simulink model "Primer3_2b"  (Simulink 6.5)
settings: Solver=ode23t  SolverMode=SingleTasking  StartTime=0.0  StopTime=0.6  RelTol=1e-3  AbsTol=1e-6
undefined symbols (not defined in the file or in its folder): blocks, Continuous, powergui, ZData
libraries: powerlib x14

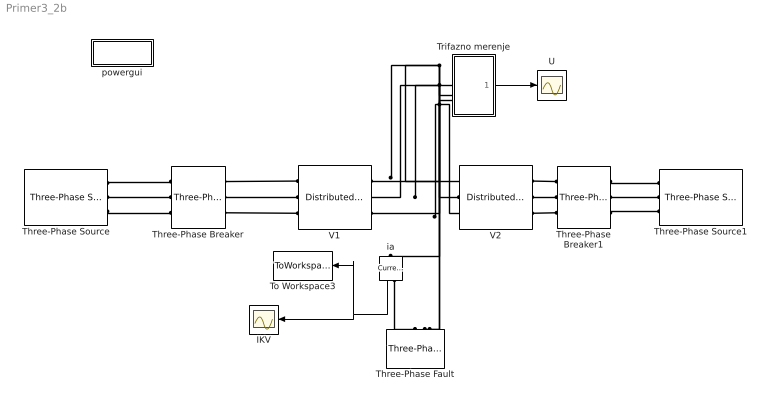
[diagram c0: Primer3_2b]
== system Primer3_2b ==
  IKV : Scope
  Three-Phase Breaker : powerlib/Elements/Three-Phase Breaker  DialogController=PMDialogs.PMDefaultMaskDlg  SystemSampleTime=-1  InitialState=closed  SwitchA=on  SwitchB=off  SwitchC=off  SwitchTimes="[ 10/50  20/50 ]"  External=off  BreakerResistance=0.001  SnubberResistance=1e6  SnubberCapacitance=inf  Measurements=None
  Three-Phase Breaker1 : powerlib/Elements/Three-Phase Breaker  Orientation=left  DialogController=PMDialogs.PMDefaultMaskDlg  SystemSampleTime=-1  InitialState=closed  SwitchA=on  SwitchB=off  SwitchC=off  SwitchTimes="[ 10/50  20/50 ]"  External=off  BreakerResistance=0.001  SnubberResistance=1e6  SnubberCapacitance=inf  Measurements=None
  Three-Phase Fault : powerlib/Elements/Three-Phase Fault  Orientation=down  DialogController=PMDialogs.PMDefaultMaskDlg  SystemSampleTime=-1  FaultA=on  FaultB=off  FaultC=off  FaultResistance=0.001  GroundFault=on  GroundResistance=0.001  External=off  SwitchStatus=[1 0]  SwitchTimes=[ 3/50 15/50]  InitialStates=[0 0 1]  SnubberResistance=1e6  SnubberCapacitance=inf  Measurements=None
  Three-Phase Source : powerlib/Electrical Sources/Three-Phase Source  DialogController=PMDialogs.PMDefaultMaskDlg  SystemSampleTime=-1  Voltage=410e3  PhaseAngle=0  Frequency=50  InternalConnection=Yg  SpecifyImpedance=on  Resistance=0.8929  Inductance=16.58e-3  ShortCircuitLevel=sqrt(3)*400e3*16e3  BaseVoltage=400e3  XRratio=10
  Three-Phase Source1 : powerlib/Electrical Sources/Three-Phase Source  Orientation=left  DialogController=PMDialogs.PMDefaultMaskDlg  SystemSampleTime=-1  Voltage=395e3  PhaseAngle=-2.5  Frequency=50  InternalConnection=Yg  SpecifyImpedance=on  Resistance=0.8929  Inductance=16.58e-3  ShortCircuitLevel=sqrt(3)*400e3*14e3  BaseVoltage=400e3  XRratio=10
  To Workspace3 : ToWorkspace  VariableName=ikv  SampleTime=-1  SaveFormat=Array
  Trifazno merenje : Subsystem
  U : Scope
  V1 : powerlib/Elements/Distributed Parameters Line  DialogController=PMDialogs.PMDefaultMaskDlg  SystemSampleTime=-1  Phases=3  Frequency=50  Resistance=[0.029983 0.29405]  Inductance=[0.0010055 0.0025377]  Capacitance=[1.1784e-008 8.6541e-009]  Length=113.5/2  x1=[0 5.31470182416808e-011 178450.018618737 -366847.020662789;5.31896283741607e-005 5.41899780765739e-011 184554.839172681 -363814.04185674;0.000106379256748321 5.5217807089294e-011 190608.12867694 -360679.479588827;0.000159568885122482 5.62302182913874e-011 196608.19694358 -357444.209085539;0.000212758513496643 5.72269289993319e-011 202553.368645001 -354109.133692926;0.000265948141870804 5.82076609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  x2=[0 -3.7359824086561e-011 172736.109706228 -365994.140775089;5.31896283741607e-005 -4.15549298166249e-011 178827.477001409 -363056.756096685;0.000106379256748321 -4.57384326585573e-011 184868.912430032 -360017.999404301;0.000159568885122482 -4.99091645026855e-011 190858.729114034 -356878.719173774;0.000212758513496643 -5.40659608052301e-011 196795.254588242 -353639.791948936;0.000265948141870804 -5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  x3=[0 6.15163419918279e-012 586.956046574621 -949.442634179271;5.31896283741607e-005 6.07772862185656e-012 602.738564141177 -939.502495741663;0.000106379256748321 6.00212603275329e-012 618.352786197114 -929.300031211689;0.000159568885122482 5.92484754148351e-012 633.794352969173 -918.838089302008;0.000212758513496643 5.84591472559994e-012 649.058952892574 -908.119591176059;0.000265948141870804 5.7653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  x4=[0 -5.27235691341477e-012 533.264836498699 -1585.21009257672;5.31896283741607e-005 -5.22831622679303e-012 559.67803894775 -1576.07833440241;0.000106379256748321 -5.18281569970079e-012 585.934969163778 -1566.50650664595;0.000159568885122482 -5.1358680367083e-012 612.028295736881 -1556.49728193482;0.000212758513496643 -5.08748634645237e-012 637.950732938252 -1546.05345502561;0.000265948141870804 -5.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  x5=0.000265948141870804  Measurements=None
  V2 : powerlib/Elements/Distributed Parameters Line  DialogController=PMDialogs.PMDefaultMaskDlg  SystemSampleTime=-1  Phases=3  Frequency=50  Resistance=[0.029983 0.29405]  Inductance=[0.0010055 0.0025377]  Capacitance=[1.1784e-008 8.6541e-009]  Length=113.5/2  x1=[0 -3.7359824086561e-011 172736.109706228 -365994.140775089;5.31896283741607e-005 -4.15549298166249e-011 178827.477001409 -363056.756096685;0.000106379256748321 -4.57384326585573e-011 184868.912430032 -360017.999404301;0.000159568885122482 -4.99091645026855e-011 190858.729114034 -356878.719173774;0.000212758513496643 -5.40659608052301e-011 196795.254588242 -353639.791948936;0.000265948141870804 -5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  x2=[0 -1.00365319719216e-010 166509.443707765 -363699.090775954;5.31896283741607e-005 -9.78077225317173e-011 172563.331767605 -360866.069344832;0.000106379256748321 -9.52228156587506e-011 178569.037023553 -357932.287579098;0.000159568885122482 -9.26113208530759e-011 184524.882574059 -354898.564643695;0.000212758513496643 -8.99739672912847e-011 190429.205439304 -351765.747608946;0.000265948141870804 -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  x3=[0 -9.13979376899358e-012 644.436346866573 -910.109116757214;5.31896283741607e-005 -9.09687067248558e-012 659.553606600837 -899.214017677193;0.000106379256748321 -9.05140756512387e-012 674.486707036846 -888.067841776699;0.000159568885122482 -9.00341714103046e-012 689.231478582818 -876.673701269678;0.000212758513496643 -8.9529127999999e-012 703.783804231807 -865.034777606277;0.000265948141870804 -8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  x4=[0 8.15651641056055e-012 435.415414146165 -1612.56297375389;5.31896283741607e-005 8.11939388275095e-012 462.299323032324 -1605.06238605293;0.000106379256748321 8.08000427328985e-012 489.05414958452 -1597.11363589828;0.000159568885122482 8.03835858046876e-012 515.672423371187 -1588.71894272478;0.000212758513496643 7.9944684325185e-012 542.146712088759 -1579.88065048263;0.000265948141870804 7.948346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  x5=0.000265948141870804  Measurements=None
  ia : powerlib/Measurements/Current Measurement  Orientation=down  DialogController=PMDialogs.PMDefaultMaskDlg  SystemSampleTime=-1  PhasorSimulation=off  OutputType=Complex  PSBequivalent=0
  powergui : Subsystem  AncestorBlock=powerlib/powergui  InitFcn=powergui( 'InitFcn_Callback' , gcb , 0 , [ ] );  mask(PSB option menu block){SimulationMode=Continuous, SampleTime=50e-6, echomessages=off, RestoreLinks=warning, x0status=blocks, Frange=[0:2:500], Ylog=off, Xlog=on, ShowGrid=off, save=off, variable=ZData, structure=, ZoomFFT=on, StartTime=0.0, cycles=1, DisplayStyle=1, fundamental=60, FreqAxis=off, MaxFrequency=1000, frequencyindice=50, frequencyindicesteady=1, RmsSteady=1, display=off, Ts=0, frequency=60, methode=off, HookPort=off, Interpol=off}
      mask prompts: SimulationMode "Simulation mode"; SampleTime "Sample time Ts (when simulation mode is Discrete) (s)"; echomessages "Echo  Messages"; RestoreLinks "Restore disabled links"; x0status "Initial electrical states status"; Frange "Impedance tool: Frequency Range"; Ylog "Impedance tool: Log impedance"; Xlog "Impedance tool: log Frequency"; ShowGrid "Impedance tool: grid"; save "Impedance tool: Save Data To Workspace"; variable "Impedance tool: Variable Name"; structure "Structure Name (PSBFFTSCOPE)"; ZoomFFT "ZoomFFT (PSBFFTSCOPE)"; StartTime "Start Time (PSBFFTSCOPE)"; cycles "Cycles (PSBFFTSCOPE)"; DisplayStyle "Display style (PSBFFTSCOPE)"; fundamental "Fundamental (PSBFFTSCOPE)"; FreqAxis "Frequency Axis (PSBFFTSCOPE)"; MaxFrequency "Max Frequency (PSBFFTSCOPE)"; frequencyindice "Load flow frequency (Hz)"; frequencyindicesteady "Frequency indice (STEADYSTATE)"; RmsSteady "RMS display (STEADYSTATE)"; display "Display Results"; Ts "OBSOLETE 1"; frequency "Phasor frequency (Hz)"; methode "Phasor simulation"; HookPort "Hook port"; Interpol "Interpolate"
      mask init:
      | powerlibroot = which('powersysdomain');
      | PSBroot = powerlibroot(1:end-16);
      | %
      | switch SimulationMode
      | 	case 1
      | 		message=sprintf('Continuous');
      | 	case 2
      |         SampleTimeeval=evalin('base',SampleTime,'NaN');
      |         if isnan(SampleTimeeval)
      |             message=sprintf('Warning !!,\nUndefined sample time');
      |         else
      |             message=sprintf('Discrete,\nTs = %.4g s.',SampleTimeeval);
      |         end
      | 	case 3
      | 		message=sprintf('Phasors');
      | end
      | if strcmp(bdroot,'powerlib')
      |   message='powergui';
      | end
      | power_initmask();
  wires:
  ia/1 -> IKV/1, To Workspace3/1
  Trifazno merenje/1(Izlez) -> U/1
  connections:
  Three-Phase Breaker/RConn1 -- V1/LConn1
  Three-Phase Source/RConn1 -- Three-Phase Breaker/LConn1
  Three-Phase Source/RConn2 -- Three-Phase Breaker/LConn2
  Three-Phase Source/RConn3 -- Three-Phase Breaker/LConn3
  V1/LConn2 -- Three-Phase Breaker/RConn2
  V1/LConn3 -- Three-Phase Breaker/RConn3
  Three-Phase Breaker1/LConn1 -- Three-Phase Source1/RConn1
  Three-Phase Breaker1/LConn2 -- Three-Phase Source1/RConn2
  Three-Phase Breaker1/LConn3 -- Three-Phase Source1/RConn3
  Trifazno merenje/LConn1 -- V2/LConn1 -- V1/RConn1 -- ia/LConn1
  Trifazno merenje/LConn2 -- V1/RConn2 -- V2/LConn2 -- Three-Phase Fault/LConn2
  Trifazno merenje/LConn3 -- V2/LConn3 -- V1/RConn3 -- Three-Phase Fault/LConn3
  Three-Phase Breaker1/RConn1 -- V2/RConn1
  V2/RConn2 -- Three-Phase Breaker1/RConn2
  V2/RConn3 -- Three-Phase Breaker1/RConn3
  ia/RConn1 -- Three-Phase Fault/LConn1

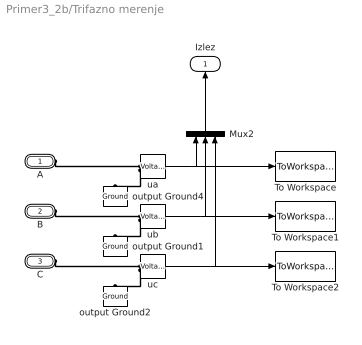
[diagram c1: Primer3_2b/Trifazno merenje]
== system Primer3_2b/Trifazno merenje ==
  Mux2 : Mux  Orientation=up  Inputs=3
  To Workspace : ToWorkspace  VariableName=ua  SampleTime=-1  SaveFormat=Array
  To Workspace1 : ToWorkspace  VariableName=ub  SampleTime=-1  SaveFormat=Array
  To Workspace2 : ToWorkspace  VariableName=uc  SampleTime=-1  SaveFormat=Array
  output Ground1 : powerlib/Elements/Ground  Orientation=down  DialogController=PMDialogs.PMDefaultMaskDlg  PhysicalDomain=powersysdomain  SubClassName=unknown  LeftPortType=p1  RightPortType=p1  LConnTagsString=a
  output Ground2 : powerlib/Elements/Ground  Orientation=down  DialogController=PMDialogs.PMDefaultMaskDlg  PhysicalDomain=powersysdomain  SubClassName=unknown  LeftPortType=p1  RightPortType=p1  LConnTagsString=a
  output Ground4 : powerlib/Elements/Ground  Orientation=down  DialogController=PMDialogs.PMDefaultMaskDlg  PhysicalDomain=powersysdomain  SubClassName=unknown  LeftPortType=p1  RightPortType=p1  LConnTagsString=a
  ua : powerlib/Measurements/Voltage Measurement  Tag=PoWeRsYsTeMmEaSuReMeNt  DialogController=PMDialogs.PMDefaultMaskDlg  SystemSampleTime=-1  PhasorSimulation=off  OutputType=Magnitude  PSBequivalent=0
  ub : powerlib/Measurements/Voltage Measurement  Tag=PoWeRsYsTeMmEaSuReMeNt  DialogController=PMDialogs.PMDefaultMaskDlg  SystemSampleTime=-1  PhasorSimulation=off  OutputType=Magnitude  PSBequivalent=0
  uc : powerlib/Measurements/Voltage Measurement  Tag=PoWeRsYsTeMmEaSuReMeNt  DialogController=PMDialogs.PMDefaultMaskDlg  SystemSampleTime=-1  PhasorSimulation=off  OutputType=Magnitude  PSBequivalent=0
  A : PMIOPort  Port=1  Side=Left
  B : PMIOPort  Port=2  Side=Left
  C : PMIOPort  Port=3  Side=Left
  Izlez : Outport  Orientation=up
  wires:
  ua/1 -> Mux2/1, To Workspace/1
  ub/1 -> Mux2/2, To Workspace1/1
  uc/1 -> Mux2/3, To Workspace2/1
  Mux2/1 -> Izlez/1
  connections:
  ub/LConn2 -- output Ground1/LConn1
  uc/LConn2 -- output Ground2/LConn1
  ua/LConn2 -- output Ground4/LConn1
  A/RConn1 -- ua/LConn1
  B/RConn1 -- ub/LConn1
  C/RConn1 -- uc/LConn1

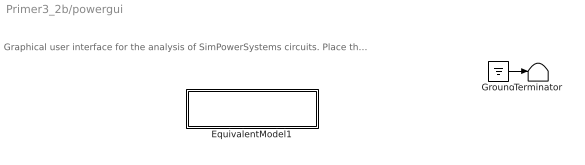
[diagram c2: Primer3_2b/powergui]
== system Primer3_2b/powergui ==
  note: Graphical user interface for the analysis of SimPowerSystems circuits. Place the Powergui block in the top-level of your model and double-click on it to open the GUI.
  EquivalentModel1 : Subsystem
  Ground : Ground
  Terminator : Terminator
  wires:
  Ground/1 -> Terminator/1

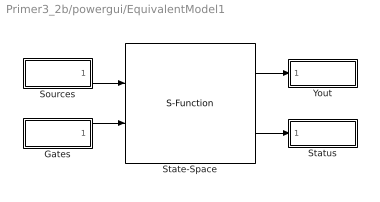
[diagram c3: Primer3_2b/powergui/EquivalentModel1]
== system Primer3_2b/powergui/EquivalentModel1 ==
  Gates : Subsystem
  Sources : Subsystem
  State-Space : S-Function  FunctionName=sfun_spssw_contc  Parameters=A, B, C, D, x0, SwitchResistance ,SwitchType, SwitchGateInitialValue, OutputsToResetToZero
  Status : Subsystem
  Yout : Subsystem
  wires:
  Gates/1(gates) -> State-Space/2
  Sources/1(u) -> State-Space/1
  State-Space/2 -> Status/1(status)
  State-Space/1 -> Yout/1(v,i)

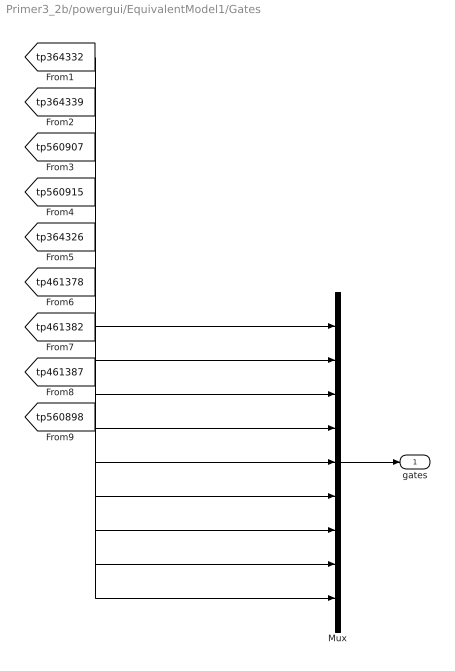
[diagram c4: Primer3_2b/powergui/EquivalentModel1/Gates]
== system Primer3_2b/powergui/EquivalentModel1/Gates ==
  Mux : Mux  Inputs=[1 1 1 1 1 1 1 1 1]
  gates : Outport
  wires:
  Mux/1 -> gates/1
  [tp364332] -> Mux/1
  [tp364339] -> Mux/2
  [tp560907] -> Mux/3
  [tp560915] -> Mux/4
  [tp364326] -> Mux/5
  [tp461378] -> Mux/6
  [tp461382] -> Mux/7
  [tp461387] -> Mux/8
  [tp560898] -> Mux/9

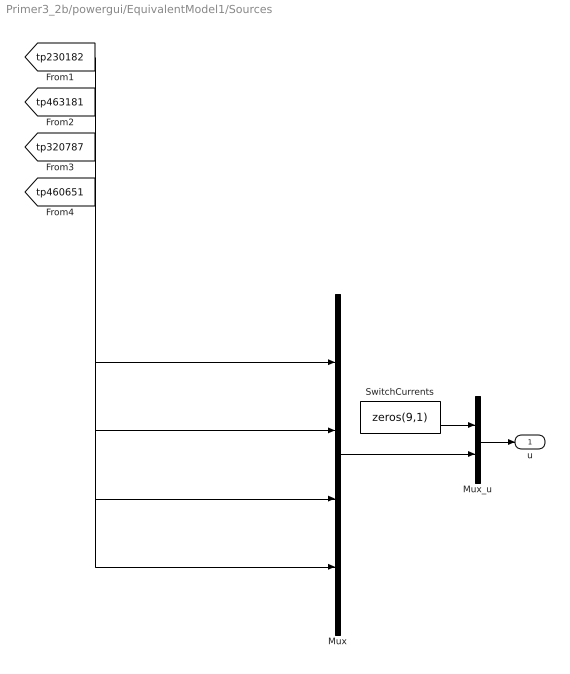
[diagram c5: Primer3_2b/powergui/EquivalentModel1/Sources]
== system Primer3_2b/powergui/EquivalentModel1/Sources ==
  Mux : Mux  Inputs=[6 6 3 3]
  Mux_u : Mux  Inputs=[9 18]
  SwitchCurrents : Constant  Value=zeros(9,1)  OutDataType=sfix(16)  ConRadixGroup=Use specified scaling  OutScaling=2^0  SampleTime=inf  FramePeriod=inf
  u : Outport
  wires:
  Mux/1 -> Mux_u/2
  SwitchCurrents/1 -> Mux_u/1
  Mux_u/1 -> u/1
  [tp230182] -> Mux/1
  [tp463181] -> Mux/2
  [tp320787] -> Mux/3
  [tp460651] -> Mux/4

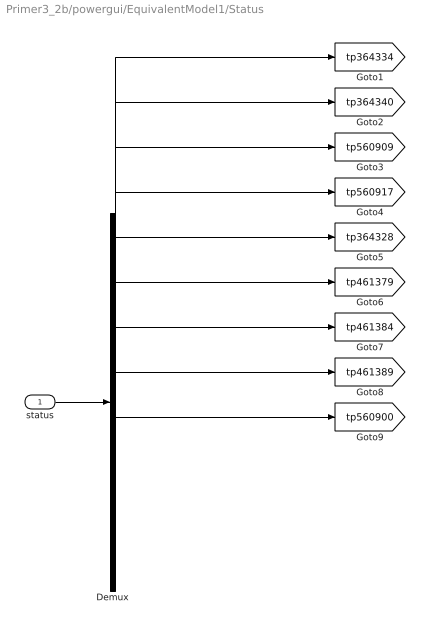
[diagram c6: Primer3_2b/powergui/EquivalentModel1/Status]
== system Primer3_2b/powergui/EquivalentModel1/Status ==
  status : Inport
  Demux : Demux  Outputs=[1 1 1 1 1 1 1 1 1]
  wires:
  status/1 -> Demux/1
  Demux/1 -> [tp364334]
  Demux/2 -> [tp364340]
  Demux/3 -> [tp560909]
  Demux/4 -> [tp560917]
  Demux/5 -> [tp364328]
  Demux/6 -> [tp461379]
  Demux/7 -> [tp461384]
  Demux/8 -> [tp461389]
  Demux/9 -> [tp560900]

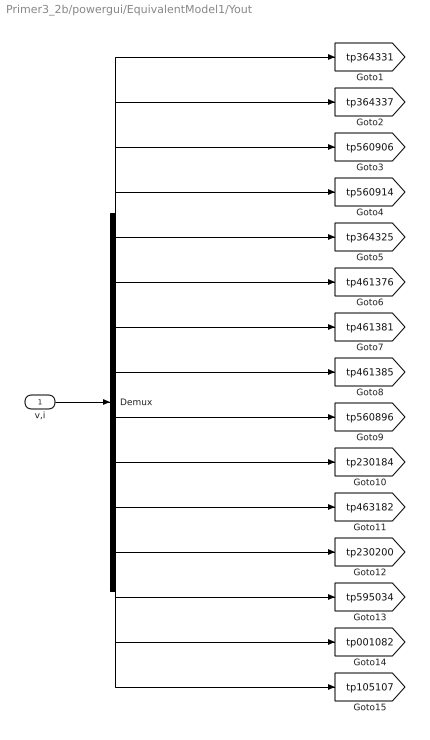
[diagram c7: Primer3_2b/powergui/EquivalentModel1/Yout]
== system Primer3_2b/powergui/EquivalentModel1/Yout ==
  v,i : Inport
  Demux : Demux  Outputs=[1 1 1 1 1 1 1 1 1 6 6 1 1 1 1]
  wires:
  v,i/1 -> Demux/1
  Demux/1 -> [tp364331]
  Demux/2 -> [tp364337]
  Demux/3 -> [tp560906]
  Demux/4 -> [tp560914]
  Demux/5 -> [tp364325]
  Demux/6 -> [tp461376]
  Demux/7 -> [tp461381]
  Demux/8 -> [tp461385]
  Demux/9 -> [tp560896]
  Demux/10 -> [tp230184]
  Demux/11 -> [tp463182]
  Demux/12 -> [tp230200]
  Demux/13 -> [tp595034]
  Demux/14 -> [tp001082]
  Demux/15 -> [tp105107]
